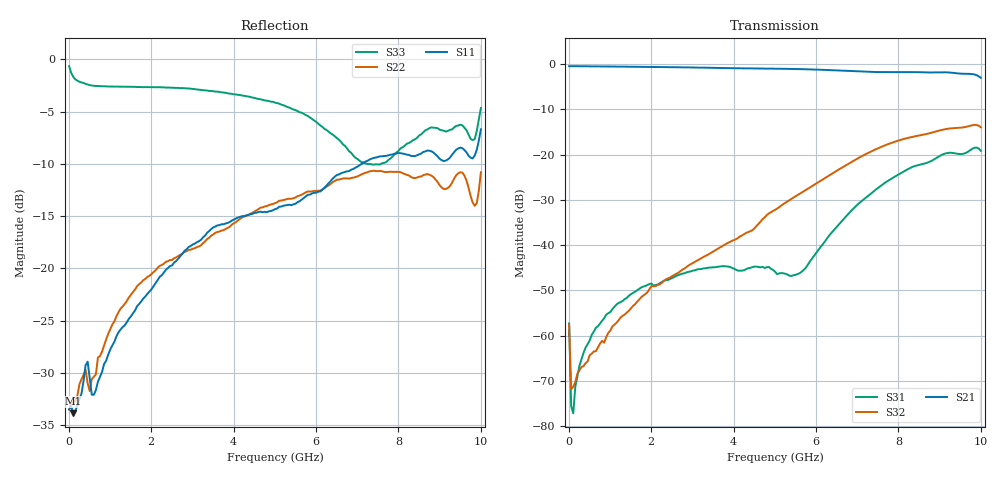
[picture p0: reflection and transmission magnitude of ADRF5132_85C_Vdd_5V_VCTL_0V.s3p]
! Device:  ADRF5132
! Description: Silicon SPDT Switch
! Frequency:  0.7 -  5 GHz
! Ports:
!	RFC	= Port 1
!	RF1	= Port 2
!  RF2  = Port 3
! Vdd:  5 Volt
! Control:  0/0 Volt
! Data:  Data was collected using a calibrated 4 port network analyzer and de-embedded using AtaiTec's In Situ De-Embedding.
! Note:  Analog Devices supplies this data as a sample of measured data
!  for this product.  Your particular data for this product may vary.
!  Data was taken at 85 degrees C.
!  Analog Devices reserves the right to change this data at anytime.
# GHZ S DB R 50.0
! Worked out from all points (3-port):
!   201 points, 10 MHz to 10 GHz, reference 50 ohm
!   strongest paths, dB at 10 MHz, 2.507 GHz, 5.005 GHz, 7.503 GHz, 10 GHz:
!     S21: -0.5, -0.7, -1.0, -1.8, -3.0
!     S32: -57.7, -46.9, -32.2, -18.6, -14.0
!     S31: -57.3, -47.3, -45.9, -27.4, -19.2
!   lowest |S11| = -33.9 dB at 109.9 MHz (marker M1), VSWR 1.04, Z = 51.9 - j0.746 ohm
!   |S11| at or under -10 dB: start of sweep to 7.108 GHz
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0.01  -33.51 19.2  -0.45 -0.2  -57.12 -60.8
      -0.46 -0.2  -33.47 22.4  -57.17 -53.6
      -57.31 -60.2  -57.70 -59.0  -0.66 -8.2
0.05995  -33.17 -11.1  -0.46 -1.0  -76.92 -35.5
         -0.46 -1.0  -32.98 -8.6  -72.68 -39.9
         -75.61 -45.5  -71.87 -36.7  -1.29 -42.5
0.1099  -33.86 -20.7  -0.46 -1.8  -75.56 29.9
        -0.46 -1.8  -32.69 -17.5  -71.11 -21.5
        -77.19 32.6  -71.31 -21.5  -1.68 -69.0
0.3097  -32.00 -36.2  -0.46 -5.0  -64.98 74.3
        -0.46 -5.0  -30.60 -34.7  -67.23 -42.2
        -65.21 69.6  -66.94 -45.8  -2.22 -128.0
0.75925  -30.36 -79.7  -0.51 -12.0  -57.48 81.3
         -0.52 -12.0  -28.39 -61.0  -61.78 -89.4
         -57.37 80.8  -61.79 -91.3  -2.57 -164.8
2.85715  -18.18 -150.3  -0.72 -44.2  -46.01 65.7
         -0.73 -44.2  -18.37 -114.3  -44.85 -163.8
         -46.04 65.6  -44.87 -163.7  -2.79 150.4
5.005  -14.34 156.5  -1.01 -76.9  -45.83 2.2
       -1.02 -76.9  -13.75 -136.3  -32.20 175.6
       -45.86 2.2  -32.23 175.6  -4.15 118.2
7.25275  -9.70 121.5  -1.70 -112.2  -29.19 176.7
         -1.71 -112.2  -10.80 -163.9  -19.68 118.7
         -29.21 176.7  -19.69 118.6  -10.03 108.5
9.6004  -8.68 70.7  -2.14 -151.3  -19.72 73.6
        -2.14 -151.3  -11.13 164.5  -13.92 39.1
        -19.75 73.6  -13.94 39.1  -6.55 99.1
10  -6.70 31.7  -3.04 -172.3  -19.15 26.3
    -3.04 -172.3  -10.80 118.2  -13.94 13.6
    -19.18 26.2  -13.96 13.6  -4.67 29.3
